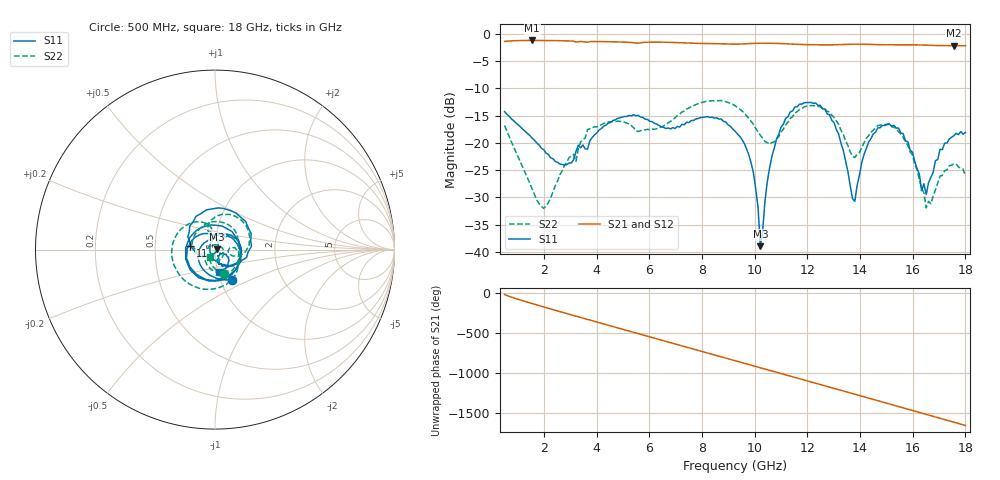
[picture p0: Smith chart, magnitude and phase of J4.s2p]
!Agilent Technologies,N5230C,MY49001096,A.09.42.15
!Agilent N5230C: A.09.42.15
!Date: Thursday, June 29, 2023 09:47:28
!Correction: S11(Full 2 Port(1,2))
!S21(Full 2 Port(1,2))
!S12(Full 2 Port(1,2))
!S22(Full 2 Port(1,2))
!S2P File: Measurements: S11, S21, S12, S22:
# Hz S  dB  R 50
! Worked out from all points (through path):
!   201 points, 500 MHz to 18 GHz, reference 50 ohm
!   highest |S21| = -1.22 dB at 1.55 GHz (marker M1); lowest = -2.2 dB at 17.56 GHz (marker M2)
!   group delay of S21, straight-line fit = 256 ps
!   lowest |S11| = -39.0 dB at 10.21 GHz (marker M3), VSWR 1.02, Z = 51.1 + j0.137 ohm
!   |S11| at or under -10 dB: start of sweep to end of sweep
!   |S22| runs from -32.0 to -12.2 dB; largest |S21 - S12| = 0.002
!   S11 on the Smith chart (normalised r, x): 500 MHz: 1.14, -0.40; 11 GHz: 0.76, +0.03; 18 GHz: 1.01, -0.25
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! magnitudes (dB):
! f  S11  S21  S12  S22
! 500 MHz  -14.3  -1.4  -1.4  -16.8
! 1.55 GHz  -19.2  -1.2  -1.2  -28.5
! 1.988 GHz  -21.3  -1.2  -1.2  -32.0
! 2.862 GHz  -24.0  -1.3  -1.3  -23.5
! 3.475 GHz  -20.4  -1.4  -1.4  -19.4
! 5.05 GHz  -15.2  -1.5  -1.5  -16.2
! 6.362 GHz  -16.8  -1.5  -1.5  -17.3
! 9.25 GHz  -17.8  -1.9  -1.9  -13.2
! 9.95 GHz  -25.5  -1.8  -1.8  -16.6
! 10.21 GHz  -39.0  -1.7  -1.7  -18.6
! 10.56 GHz  -24.6  -1.7  -1.7  -20.3
! 11 GHz  -17.1  -1.8  -1.8  -18.0
! 12.22 GHz  -12.8  -2.0  -2.0  -13.2
! 13.01 GHz  -16.3  -2.0  -2.0  -15.3
! 13.8 GHz  -30.7  -1.9  -1.9  -22.7
! 14.32 GHz  -19.9  -1.9  -1.9  -18.7
! 15.11 GHz  -16.6  -2.0  -2.0  -16.5
! 15.99 GHz  -21.7  -2.0  -2.0  -22.2
! 16.51 GHz  -29.5  -2.1  -2.1  -31.9
! 17.04 GHz  -21.2  -2.2  -2.2  -26.1
! 17.56 GHz  -18.7  -2.2  -2.2  -23.8
! 18 GHz  -18.1  -2.2  -2.2  -26.1
